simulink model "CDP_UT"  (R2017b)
settings: Solver=FixedStepDiscrete  StartTime=0.0  StopTime=10.0  FixedStep=0.01  RelTol=1e-3  EnableMultiTasking=on
undefined symbols (not defined in the file): ASWTYPE_FALSE, ASWTYPE_TRUE, CaCDP_CellTempNTCVoltTable_mV, CaCDP_CellTempTable_C, CaCDP_CMUPCBTempNTCVoltTable_mV, CaCDP_CMUPCBTempTable_C, CbCDP_DiffBusbarTempStateCheck_flg, CbCDP_DiffCellTempStateCheck_flg, CbCDP_DiffCellVoltStateCheck_flg, CbCDP_IgnorUpdateVld_flg, CbCDP_MaxBusbarTempStateCheck_flg, CbCDP_MaxCellTempStateCheck_flg, CbCDP_MaxCellVoltStateCheck_flg, CbCDP_MinBusbarTempStateCheck_flg, CbCDP_MinCellTempStateCheck_flg, CbCDP_MinCellVoltStateCheck_flg, CcCDP_AFETempConfig_numb, CcCDP_AFETempFltThd_C, CcCDP_AFETempFltThdHys_C, CcCDP_BusbarTempRngFltHiThrd_C, CcCDP_BusbarTempRngFltLowThrd_C, CcCDP_CellDiffFltLevel1_mV, CcCDP_CellDiffFltLevel2_mV, CcCDP_CellDiffFltLevel3_mV, CcCDP_CellTempLowerLimit_C, CcCDP_CellTempRngFltHiThrd_C, CcCDP_CellTempRngFltLowThrd_C, CcCDP_CellTempUpperLimit_C, CcCDP_CellVoltConfig_numb, CcCDP_CellVoltLowerLimit_mV, CcCDP_CellVoltRngHiThrd_mV, CcCDP_CellVoltRngLowThrd_mV, CcCDP_CellVoltUpdateThrd_numb, CcCDP_CellVoltUpperLimit_mV, CcCDP_ChrgMaxCellTempFltLv1Thrd_C, CcCDP_ChrgMaxCellTempFltLv2Thrd_C, CcCDP_ChrgMaxCellTempFltLv3Thrd_C, CcCDP_ChrgMaxCellTempReturnDiff_C, CcCDP_ChrgMinCellTempFltLv1Thrd_C, CcCDP_ChrgMinCellTempFltLv2Thrd_C, CcCDP_ChrgMinCellTempFltLv3Thrd_C, CcCDP_ChrgMinCellTempReturnDiff_C, CcCDP_CMUPCBTempConfig_numb, CcCDP_CMUPCBTempFltThd_C, CcCDP_CMUPCBTempFltThdHys_C, CcCDP_DiffBusbarTempFltLevel1Thrd_C, CcCDP_DiffBusbarTempFltLevel2Thrd_C, CcCDP_DiffBusbarTempReturnDifference_C, CcCDP_DiffCellTempFltLevel1Thrd_C, CcCDP_DiffCellTempFltLevel2Thrd_C, CcCDP_DiffCellTempReturnDifference_C, CcCDP_DiffCellVoltReturnDifference_mV, CcCDP_DiffVoltCheckMaxCellTempCondition_C, CcCDP_DiffVoltCheckMaxCellVoltCondition_mV, CcCDP_DiffVoltCheckMinCellTempCondition_C, CcCDP_DiffVoltCheckMinCellVoltCondition_mV, CcCDP_DiffVoltCheckPackCurrCondition_A, CcCDP_MaxAFETempIniVal_C, CcCDP_MaxBusbarTempFltLevel1Thrd_C, CcCDP_MaxBusbarTempFltLevel2Thrd_C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
libraries: AIWAYS_Powertrain_BMS_lib x148, simulink x8
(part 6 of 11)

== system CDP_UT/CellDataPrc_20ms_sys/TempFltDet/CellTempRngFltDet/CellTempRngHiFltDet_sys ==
  LbCDP_CellTempRngHiChk_flg : Inport
  GcCDP_MaxCellTemp_C : Inport  Port=2
  CDP_GbCDP_ChrgMaxCellVoltFltLv1_flg : AIWAYS_Powertrain_BMS_lib/Signals/OverWrite  OverWrite_Value=CbCDP_CellTempRngHiFltOvr_flg  OverWrite_flag=CbCDP_CellTempRngHiFltOvrSwt_flg
  Constant : Constant  Value=CcCDP_CellTempRngFltHiThrd_C
  Logical Operator1 : Logic  AllPortsSameDT=off  OutDataTypeStr=boolean
  Relational Operator : RelationalOperator  OutDataTypeStr=boolean
  LbCDP_CellTempRngHiFlt_flg : Outport
  GbCDP_CellTempRngHiFlt_flg : Outport  Port=2
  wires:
  GcCDP_MaxCellTemp_C/1 -> Relational Operator/1
  Constant/1 -> Relational Operator/2
  CDP_GbCDP_ChrgMaxCellVoltFltLv1_flg/1 -> GbCDP_CellTempRngHiFlt_flg/1  "GbCDP_CellTempRngHiFlt_flg"
  Logical Operator1/1 -> LbCDP_CellTempRngHiFlt_flg/1, CDP_GbCDP_ChrgMaxCellVoltFltLv1_flg/1  "LbCDP_CellTempRngHiFlt_flg"
  Relational Operator/1 -> Logical Operator1/2
  LbCDP_CellTempRngHiChk_flg/1 -> Logical Operator1/1

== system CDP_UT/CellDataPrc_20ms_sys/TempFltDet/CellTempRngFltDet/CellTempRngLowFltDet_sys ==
  LbCDP_CellTempRngLowChk_flg : Inport
  GcCDP_MinCellTemp_C : Inport  Port=2
  CDP_GbCDP_ChrgMaxCellVoltFltLv1_flg : AIWAYS_Powertrain_BMS_lib/Signals/OverWrite  OverWrite_Value=CbCDP_CellTempRngLowFltOvr_flg  OverWrite_flag=CbCDP_CellTempRngLowFltOvrSwt_flg
  Comparison3 : RelationalOperator  Operator=<=  OutDataTypeStr=boolean
  Constant1 : Constant  Value=CcCDP_CellTempRngFltLowThrd_C
  Logical Operator1 : Logic  AllPortsSameDT=off  OutDataTypeStr=boolean
  LbCDP_CellTempRngLowFlt_flg : Outport
  GbCDP_CellTempRngLowFlt_flg : Outport  Port=2
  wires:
  GcCDP_MinCellTemp_C/1 -> Comparison3/1
  Constant1/1 -> Comparison3/2
  Logical Operator1/1 -> CDP_GbCDP_ChrgMaxCellVoltFltLv1_flg/1, LbCDP_CellTempRngLowFlt_flg/1  "LbCDP_CellTempRngLowFlt_flg"
  CDP_GbCDP_ChrgMaxCellVoltFltLv1_flg/1 -> GbCDP_CellTempRngLowFlt_flg/1  "GbCDP_CellTempRngLowFlt_flg"
  Comparison3/1 -> Logical Operator1/2
  LbCDP_CellTempRngLowChk_flg/1 -> Logical Operator1/1

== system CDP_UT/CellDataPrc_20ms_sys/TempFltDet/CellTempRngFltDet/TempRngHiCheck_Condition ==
  LbCDP_AnyCellTempVld_flg : Inport
  Constant : Constant  Value=ASWTYPE_TRUE
  Constant1 : Constant  Value=CbCDP_MaxCellTempStateCheck_flg
  Constant2 : Constant  Value=ASWTYPE_TRUE
  Logical Operator : Logic  AllPortsSameDT=off  OutDataTypeStr=boolean
  Relational Operator : RelationalOperator  Operator===  OutDataTypeStr=boolean
  Relational Operator1 : RelationalOperator  Operator===  OutDataTypeStr=boolean
  LbCDP_CellTempRngHiChk_flg : Outport
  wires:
  Constant1/1 -> Relational Operator1/1
  Logical Operator/1 -> LbCDP_CellTempRngHiChk_flg/1  "LbCDP_CellTempRngHiChk_flg"
  Relational Operator/1 -> Logical Operator/1
  Constant2/1 -> Relational Operator1/2
  Relational Operator1/1 -> Logical Operator/2
  Constant/1 -> Relational Operator/2
  LbCDP_AnyCellTempVld_flg/1 -> Relational Operator/1

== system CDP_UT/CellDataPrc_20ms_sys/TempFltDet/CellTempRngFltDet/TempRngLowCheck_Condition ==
  LbCDP_AnyCellTempVld_flg : Inport
  Constant : Constant  Value=ASWTYPE_TRUE
  Constant3 : Constant  Value=CbCDP_MinCellTempStateCheck_flg
  Constant4 : Constant  Value=ASWTYPE_TRUE
  Logical Operator : Logic  AllPortsSameDT=off  OutDataTypeStr=boolean
  Relational Operator : RelationalOperator  Operator===  OutDataTypeStr=boolean
  Relational Operator2 : RelationalOperator  Operator===  OutDataTypeStr=boolean
  LbCDP_CellTempRngLowChk_flg : Outport
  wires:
  Relational Operator2/1 -> Logical Operator/2
  Constant3/1 -> Relational Operator2/1
  Constant4/1 -> Relational Operator2/2
  LbCDP_AnyCellTempVld_flg/1 -> Relational Operator/1
  Constant/1 -> Relational Operator/2
  Relational Operator/1 -> Logical Operator/1
  Logical Operator/1 -> LbCDP_CellTempRngLowChk_flg/1  "LbCDP_CellTempRngLowChk_flg"

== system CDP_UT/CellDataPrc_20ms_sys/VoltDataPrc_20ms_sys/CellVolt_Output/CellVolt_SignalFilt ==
  LaCDP_CellVolt_mV : Inport
  LaCDP_CellVoltUpdateVld_flg : Inport  Port=2
  GeUDS_CapSel_enum : Inport  Port=3
  GcUDS_CellVoltNum_numb : Inport  Port=4
  1D_Config_Word : AIWAYS_Powertrain_BMS_lib/Signals/1D_Config_Word  Default_CalPar_Name=CcCDP_CATL203CellVoltFilCfig_numb  CATL153Ah_CalPar_Name=CcCDP_CATL177CellVoltFilCfig_numb  CATL180Ah_CalPar_Name=CcCDP_CATL177CellVoltFilCfig_numb  CATL177Ah_CalPar_Name=CcCDP_CATL177CellVoltFilCfig_numb  CATL203Ah_CalPar_Name=CcCDP_CATL203CellVoltFilCfig_numb  CATL51Ah_CalPar_Name=CcCDP_CATL177CellVoltFilCfig_numb  CATL132Ah_CalPar_Name=CcCDP_CATL177CellVoltFilCfig_numb  XWD75Ah_CalPar_Name=CcCDP_CATL177CellVoltFilCfig_numb  TFE177Ah_CalPar_Name=CcCDP_CATL177CellVoltFilCfig_numb  CATLCTP248Ah_CalPar_Name=CcCDP_CATL177CellVoltFilCfig_numb
  Comparison1 : RelationalOperator  Operator===  OutDataTypeStr=boolean
  Constant2 : Constant  Value=ASWTYPE_FALSE
  InputValueCalc : Stateflow chart  TreatAsAtomicUnit=on
  MaxValue_sort : Stateflow chart  TreatAsAtomicUnit=on
  OverWrite : AIWAYS_Powertrain_BMS_lib/Signals/OverWrite  OverWrite_Value=CaCDP_CellVoltOvr_mV  OverWrite_flag=CbCDP_CellVoltOvrSwt_flg
  SignalDelay1 : Subsystem  Commented=on
  Terminator : Terminator
  Unit Delay21 : UnitDelay  SampleTime=-1  StateName=StateName
  GaCDP_CellVolt_mV : Outport
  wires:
  Unit Delay21/1 -> InputValueCalc/4(Old_Value)
  LaCDP_CellVolt_mV/1 -> InputValueCalc/1(Input_Value)
  MaxValue_sort/2(TargetOutput_Value) -> OverWrite/1
  1D_Config_Word/1 -> MaxValue_sort/2(Input_dim)
  InputValueCalc/1(Output_Value) -> Unit Delay21/1, MaxValue_sort/1(Input_Value)
  GeUDS_CapSel_enum/1 -> 1D_Config_Word/1
  LaCDP_CellVoltUpdateVld_flg/1 -> Comparison1/1
  MaxValue_sort/1(Output_Value) -> Terminator/1
  GcUDS_CellVoltNum_numb/1 -> MaxValue_sort/3(Input_num), InputValueCalc/3(Input_num)
  OverWrite/1 -> GaCDP_CellVolt_mV/1  "GaCDP_CellVolt_mV"
  Constant2/1 -> Comparison1/2
  Comparison1/1 -> InputValueCalc/2(Update)  "LaCDP_CellVoltUpdateVld_flg"

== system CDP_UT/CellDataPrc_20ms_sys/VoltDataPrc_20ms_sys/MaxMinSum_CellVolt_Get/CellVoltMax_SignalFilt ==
  LcCDP_MaxCellVolt_mV : Inport
  LcCDP_MaxCellVoltNumb_numb : Inport  Port=2
  LbCDP_CellVoltUpdateVld_flg : Inport  Port=3
  GeUDS_CapSel_enum : Inport  Port=4
  1D_Config_Word : AIWAYS_Powertrain_BMS_lib/Signals/1D_Config_Word  Default_CalPar_Name=CcCDP_CATL203MaxCellVoltFilCfig_numb  CATL153Ah_CalPar_Name=CcCDP_CATL177MaxCellVoltFilCfig_numb  CATL180Ah_CalPar_Name=CcCDP_CATL177MaxCellVoltFilCfig_numb  CATL177Ah_CalPar_Name=CcCDP_CATL177MaxCellVoltFilCfig_numb  CATL203Ah_CalPar_Name=CcCDP_CATL203MaxCellVoltFilCfig_numb  CATL51Ah_CalPar_Name=CcCDP_CATL177MaxCellVoltFilCfig_numb  CATL132Ah_CalPar_Name=CcCDP_CATL177MaxCellVoltFilCfig_numb  XWD75Ah_CalPar_Name=CcCDP_CATL177MaxCellVoltFilCfig_numb  TFE177Ah_CalPar_Name=CcCDP_CATL177MaxCellVoltFilCfig_numb  CATLCTP248Ah_CalPar_Name=CcCDP_CATL177MaxCellVoltFilCfig_numb
  InputValueCalc : Stateflow chart  TreatAsAtomicUnit=on
  MaxValue_sort : Stateflow chart  TreatAsAtomicUnit=on
  SignalDelay1 : Subsystem  Commented=on
  Unit Delay21 : UnitDelay  SampleTime=-1  StateName=StateName
  ValueCalc : Subsystem
  ValueIndexCalc : Subsystem
  GcCDP_MaxCellVolt_mV : Outport
  GcCDP_MaxCellVoltNumb_numb : Outport  Port=2
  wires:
  ValueCalc/2(Output_index1) -> ValueIndexCalc/1(Output_index1)
  MaxValue_sort/2(Output_index) -> ValueCalc/2(Output_index)
  MaxValue_sort/1(Output_Value) -> ValueCalc/1(Output_Value)
  Unit Delay21/1 -> InputValueCalc/3(Old_Value)
  LcCDP_MaxCellVolt_mV/1 -> InputValueCalc/1(Input_Value)
  LcCDP_MaxCellVoltNumb_numb/1 -> ValueIndexCalc/2(LcCDP_MaxCellVoltNumb_numb)
  ValueIndexCalc/1(GcCDP_MaxCellVoltNumb_numb) -> GcCDP_MaxCellVoltNumb_numb/1
  ValueCalc/1(GcCDP_MaxCellVolt_mV) -> GcCDP_MaxCellVolt_mV/1
  1D_Config_Word/1 -> MaxValue_sort/2(Input_dim), ValueCalc/3(CcCDP_CellVoltFilConfig_numb)
  InputValueCalc/1(Output_Value) -> MaxValue_sort/1(Input_Value), Unit Delay21/1
  GeUDS_CapSel_enum/1 -> 1D_Config_Word/1
  LbCDP_CellVoltUpdateVld_flg/1 -> ValueIndexCalc/3(LbCDP_CellVoltUpdateVld_flg), InputValueCalc/2(Rige)

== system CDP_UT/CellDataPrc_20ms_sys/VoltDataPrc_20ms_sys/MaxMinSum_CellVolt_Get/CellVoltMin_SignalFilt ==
  GeUDS_CapSel_enum : Inport
  LbCDP_CellVoltUpdateVld_flg : Inport  Port=2
  LcCDP_MinCellVolt_mV : Inport  Port=3
  LcCDP_MinCellVoltNumb_numb : Inport  Port=4
  1D_Config_Word : AIWAYS_Powertrain_BMS_lib/Signals/1D_Config_Word  Default_CalPar_Name=CcCDP_CATL203MaxCellVoltFilCfig_numb  CATL153Ah_CalPar_Name=CcCDP_CATL177MaxCellVoltFilCfig_numb  CATL180Ah_CalPar_Name=CcCDP_CATL177MaxCellVoltFilCfig_numb  CATL177Ah_CalPar_Name=CcCDP_CATL177MaxCellVoltFilCfig_numb  CATL203Ah_CalPar_Name=CcCDP_CATL203MaxCellVoltFilCfig_numb  CATL51Ah_CalPar_Name=CcCDP_CATL177MaxCellVoltFilCfig_numb  CATL132Ah_CalPar_Name=CcCDP_CATL177MaxCellVoltFilCfig_numb  XWD75Ah_CalPar_Name=CcCDP_CATL177MaxCellVoltFilCfig_numb  TFE177Ah_CalPar_Name=CcCDP_CATL177MaxCellVoltFilCfig_numb  CATLCTP248Ah_CalPar_Name=CcCDP_CATL177MaxCellVoltFilCfig_numb
  Data Type Conversion : DataTypeConversion
  Data Type Conversion1 : DataTypeConversion
  InputValueCalc : Stateflow chart  TreatAsAtomicUnit=on
  MinValue_sort : Stateflow chart  TreatAsAtomicUnit=on
  SignalDelay1 : Subsystem  Commented=on
  Unit Delay21 : UnitDelay  SampleTime=-1  StateName=StateName
  ValueCalc : Subsystem
  ValueIndexCalc : Subsystem
  GcCDP_MinCellVolt_mV : Outport
  GcCDP_MinCellVoltNumb_numb : Outport  Port=2
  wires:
  1D_Config_Word/1 -> ValueCalc/3(CcCDP_CellVoltFilConfig_numb), Data Type Conversion/1
  GeUDS_CapSel_enum/1 -> 1D_Config_Word/1
  Data Type Conversion1/1 -> MinValue_sort/1(Input_Value)
  Data Type Conversion/1 -> MinValue_sort/2(Input_dim)
  ValueCalc/1(GcCDP_MinCellVolt_mV) -> GcCDP_MinCellVolt_mV/1
  ValueIndexCalc/1(GcCDP_MinCellVoltNumb_numb) -> GcCDP_MinCellVoltNumb_numb/1
  InputValueCalc/1(Output_Value) -> Unit Delay21/1, Data Type Conversion1/1
  LcCDP_MinCellVoltNumb_numb/1 -> ValueIndexCalc/2(LcCDP_MinCellVoltNumb_numb)
  LcCDP_MinCellVolt_mV/1 -> InputValueCalc/1(Input_Value)
  Unit Delay21/1 -> InputValueCalc/3(Old_Value)
  MinValue_sort/1(Output_Value) -> ValueCalc/1(Output_Value)
  MinValue_sort/2(Output_index) -> ValueCalc/2(Output_index)
  ValueCalc/2(Output_index1) -> ValueIndexCalc/1(Output_index1)
  LbCDP_CellVoltUpdateVld_flg/1 -> ValueIndexCalc/3(LbCDP_CellVoltUpdateVld_flg), InputValueCalc/2(Rige)

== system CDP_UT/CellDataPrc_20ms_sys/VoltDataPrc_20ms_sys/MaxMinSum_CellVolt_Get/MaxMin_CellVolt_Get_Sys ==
  LaCDP_CellVoltVld_flg : Inport
  GaISP_CellVoltUpdCnt_numb : Inport  Port=2
  LaCDP_CellVolt_mV : Inport  Port=3
  Enable : EnablePort  StatesWhenEnabling=reset
  Comparison4 : RelationalOperator  Operator===  OutDataTypeStr=boolean
  Constant1 : Constant  Value=CDP_CONST0_NUMB
  Constant2 : Constant  Value=CbCDP_IgnorUpdateVld_flg
  Constant3 : Constant  Value=CcCDP_CellVoltConfig_numb
  Logical : Logic  OutDataTypeStr=boolean
  MaxMin_CellVolt_ForIterator : Subsystem
  Switch : Switch  Criteria=u2 ~= 0  Threshold=1  RndMeth=Zero
  LcCDP_MaxCellVolt_mV : Outport
  LcCDP_MaxCellVoltNumb_numb : Outport  Port=2
  LcCDP_MinCellVolt_mV : Outport  Port=3
  LcCDP_MinCellVoltNumb_numb : Outport  Port=4
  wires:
  LaCDP_CellVolt_mV/1 -> MaxMin_CellVolt_ForIterator/2(LaCDP_CellVolt_mV)
  Constant3/1 -> MaxMin_CellVolt_ForIterator/1(CcCDP_CellVoltConfig_numb)  "CcCDP_CellVoltConfig_numb"
  MaxMin_CellVolt_ForIterator/2(LcCDP_MaxCellVoltNumb_numb) -> LcCDP_MaxCellVoltNumb_numb/1  "LcCDP_MaxCellVoltNumb_numb"
  MaxMin_CellVolt_ForIterator/1(LcCDP_MaxCellVolt_mV) -> LcCDP_MaxCellVolt_mV/1  "LcCDP_MaxCellVolt_mV"
  MaxMin_CellVolt_ForIterator/3(LcCDP_MinCellVolt_mV) -> LcCDP_MinCellVolt_mV/1  "LcCDP_MinCellVolt_mV"
  MaxMin_CellVolt_ForIterator/4(LcCDP_MinCellVoltNumb_numb) -> LcCDP_MinCellVoltNumb_numb/1  "LcCDP_MinCellVoltNumb_numb"
  Comparison4/1 -> Logical/2
  LaCDP_CellVoltVld_flg/1 -> Logical/1, Switch/1
  Logical/1 -> Switch/3
  Constant2/1 -> Switch/2
  Constant1/1 -> Comparison4/2
  GaISP_CellVoltUpdCnt_numb/1 -> Comparison4/1
  Switch/1 -> MaxMin_CellVolt_ForIterator/3(LaCDP_CellVoltVld_flg)

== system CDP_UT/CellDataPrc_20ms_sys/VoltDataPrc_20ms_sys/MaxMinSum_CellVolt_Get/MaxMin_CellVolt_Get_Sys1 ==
  LaCDP_CellVoltVld_flg : Inport
  LaCDP_CellVolt_mV : Inport  Port=2
  Enable : EnablePort  StatesWhenEnabling=reset
  Constant3 : Constant  Value=CcCDP_CellVoltConfig_numb
  MaxMin_CellVolt_ForIterator : Subsystem
  OverWrite : AIWAYS_Powertrain_BMS_lib/Signals/OverWrite  OverWrite_Value=CcCDP_MaxCellVoltOvr_mV  OverWrite_flag=CbCDP_MaxCellVoltOvrSwt_flg
  OverWrite1 : AIWAYS_Powertrain_BMS_lib/Signals/OverWrite  OverWrite_Value=CcCDP_MaxCellVoltNumbOvr_numb  OverWrite_flag=CbCDP_MaxCellVoltNumbOvrSwt_flg
  OverWrite2 : AIWAYS_Powertrain_BMS_lib/Signals/OverWrite  OverWrite_Value=CcCDP_MinCellVoltOvr_mV  OverWrite_flag=CbCDP_MinCellVoltOvrSwt_flg
  OverWrite3 : AIWAYS_Powertrain_BMS_lib/Signals/OverWrite  OverWrite_Value=CcCDP_MinCellVoltNumbOvr_numb  OverWrite_flag=CbCDP_MinCellVoltNumbOvrSwt_flg
  GcCDP_MaxCellVolt_mV : Outport
  GcCDP_MaxCellVoltNumb_numb : Outport  Port=2
  GcCDP_MinCellVolt_mV : Outport  Port=3
  GcCDP_MinCellVoltNumb_numb : Outport  Port=4
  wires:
  LaCDP_CellVoltVld_flg/1 -> MaxMin_CellVolt_ForIterator/3(LaCDP_CellVoltVld_flg)
  MaxMin_CellVolt_ForIterator/4(LcCDP_MinCellVoltNumb_numb) -> OverWrite3/1
  MaxMin_CellVolt_ForIterator/3(LcCDP_MinCellVolt_mV) -> OverWrite2/1
  MaxMin_CellVolt_ForIterator/2(LcCDP_MaxCellVoltNumb_numb) -> OverWrite1/1
  MaxMin_CellVolt_ForIterator/1(LcCDP_MaxCellVolt_mV) -> OverWrite/1
  OverWrite3/1 -> GcCDP_MinCellVoltNumb_numb/1  "GcCDP_MinCellVoltNumb_numb"
  OverWrite2/1 -> GcCDP_MinCellVolt_mV/1  "GcCDP_MinCellVolt_mV"
  OverWrite/1 -> GcCDP_MaxCellVolt_mV/1  "GcCDP_MaxCellVolt_mV"
  OverWrite1/1 -> GcCDP_MaxCellVoltNumb_numb/1  "GcCDP_MaxCellVoltNumb_numb"
  Constant3/1 -> MaxMin_CellVolt_ForIterator/1(CcCDP_CellVoltConfig_numb)  "CcCDP_CellVoltConfig_numb"
  LaCDP_CellVolt_mV/1 -> MaxMin_CellVolt_ForIterator/2(LaCDP_CellVolt_mV)

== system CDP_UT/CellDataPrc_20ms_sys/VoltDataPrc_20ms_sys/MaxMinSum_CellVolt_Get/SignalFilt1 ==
  Input_Value : Inport
  Input_Numb : Inport  Port=2
  GeUDS_CapSel_enum : Inport  Port=3
  1D_Config_Word : AIWAYS_Powertrain_BMS_lib/Signals/1D_Config_Word  Default_CalPar_Name=CcCDP_CATL203CellVoltFilConfig_numb  CATL153Ah_CalPar_Name=CcCDP_CATL177CellVoltFilConfig_numb  CATL180Ah_CalPar_Name=CcCDP_CATL177CellVoltFilConfig_numb  CATL177Ah_CalPar_Name=CcCDP_CATL177CellVoltFilConfig_numb  CATL203Ah_CalPar_Name=CcCDP_CATL203CellVoltFilConfig_numb  CATL51Ah_CalPar_Name=CcCDP_CATL177CellVoltFilConfig_numb  CATL132Ah_CalPar_Name=CcCDP_CATL177CellVoltFilConfig_numb  XWD75Ah_CalPar_Name=CcCDP_CATL177CellVoltFilConfig_numb  TFE177Ah_CalPar_Name=CcCDP_CATL177CellVoltFilConfig_numb  CATLCTP248Ah_CalPar_Name=CcCDP_CATL177CellVoltFilConfig_numb
  Constant2 : Constant  Value=CDP_CONST1_NUMB
  Constant4 : Constant  Value=CDP_CONST2_NUMB
  Constant6 : Constant  Value=CDP_CONST1_NUMB
  Constant7 : Constant  Value=CDP_CONST2_NUMB
  Data Type Conversion : DataTypeConversion
  Data Type Conversion1 : DataTypeConversion
  MaxCellVolt_sort : Stateflow chart  TreatAsAtomicUnit=on
  Product1 : Product  Inputs=*/  OutDataTypeStr=Inherit: Inherit via back propagation
  Product2 : Product  Inputs=*/  OutDataTypeStr=Inherit: Inherit via back propagation
  Selector : Selector  InputPortWidth=5  IndexOptions=Index vector (port)  Indices=[1 3]  OutputSizes=1
  Selector1 : Selector  InputPortWidth=5  IndexOptions=Index vector (port)  Indices=[1 3]  OutputSizes=1
  Selector2 : Selector  IndexMode=Zero-based  InputPortWidth=5  IndexOptions=Index vector (port)  Indices=[1 3]  OutputSizes=1
  SignalDelay1 : Subsystem
  SignalDelay2 : Subsystem
  Sum : Sum  OutDataTypeStr=Inherit: Inherit via back propagation  RndMeth=Zero
  Sum1 : Sum  OutDataTypeStr=Inherit: Inherit via back propagation  RndMeth=Zero
  Output_Value : Outport
  Output_Numb : Outport  Port=2
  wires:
  Input_Value/1 -> SignalDelay1/1(u)
  Input_Numb/1 -> SignalDelay2/1(u)
  SignalDelay1/1(y) -> Data Type Conversion1/1
  MaxCellVolt_sort/1(Output_Value) -> Selector/1
  [CcCDP_CellVoltFilConfig_numb] -> Sum/1
  Constant2/1 -> Sum/2
  Sum/1 -> Product1/1
  Constant4/1 -> Product1/2
  Product1/1 -> Selector/2
  Product2/1 -> Selector1/2
  Constant7/1 -> Product2/2
  Sum1/1 -> Product2/1
  Constant6/1 -> Sum1/2
  [CcCDP_CellVoltFilConfig_numb] -> Sum1/1
  MaxCellVolt_sort/2(Output_index) -> Selector1/1
  SignalDelay2/1(y) -> Selector2/1
  Selector1/1 -> Selector2/2
  Selector2/1 -> Output_Numb/1
  Selector/1 -> Output_Value/1
  Data Type Conversion/1 -> MaxCellVolt_sort/2(Input_dim)
  Data Type Conversion1/1 -> MaxCellVolt_sort/1(Input_Value)
  GeUDS_CapSel_enum/1 -> 1D_Config_Word/1
  1D_Config_Word/1 -> Data Type Conversion/1, [CcCDP_CellVoltFilConfig_numb]

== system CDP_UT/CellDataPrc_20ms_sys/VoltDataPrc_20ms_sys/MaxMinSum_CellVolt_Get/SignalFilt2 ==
  Input_Value : Inport
  Input_Numb : Inport  Port=2
  GeUDS_CapSel_enum : Inport  Port=3
  InputValueVld : Inport  Port=4
  InputValueUpdate : Inport  Port=5
  1D_Config_Word : AIWAYS_Powertrain_BMS_lib/Signals/1D_Config_Word  Default_CalPar_Name=CcCDP_CATL203CellVoltFilConfig_numb  CATL153Ah_CalPar_Name=CcCDP_CATL177CellVoltFilConfig_numb  CATL180Ah_CalPar_Name=CcCDP_CATL177CellVoltFilConfig_numb  CATL177Ah_CalPar_Name=CcCDP_CATL177CellVoltFilConfig_numb  CATL203Ah_CalPar_Name=CcCDP_CATL203CellVoltFilConfig_numb  CATL51Ah_CalPar_Name=CcCDP_CATL177CellVoltFilConfig_numb  CATL132Ah_CalPar_Name=CcCDP_CATL177CellVoltFilConfig_numb  XWD75Ah_CalPar_Name=CcCDP_CATL177CellVoltFilConfig_numb  TFE177Ah_CalPar_Name=CcCDP_CATL177CellVoltFilConfig_numb  CATLCTP248Ah_CalPar_Name=CcCDP_CATL177CellVoltFilConfig_numb
  Bus Creator : BusCreator  Inputs=2
  Bus Selector : BusSelector  OutputSignals=signal1,signal2
  Bus Selector1 : BusSelector  OutputSignals=signal1,signal2
  Comparison4 : RelationalOperator  Operator===  OutDataTypeStr=boolean
  Constant1 : Constant  Value=CDP_CONST0_NUMB
  Data Type Conversion : DataTypeConversion
  Data Type Conversion1 : DataTypeConversion
  EdgeBi : AIWAYS_Powertrain_BMS_lib/Logical Operators/EdgeBi
  InputValueCalc : Stateflow chart  TreatAsAtomicUnit=on
  Logical : Logic  OutDataTypeStr=boolean
  MaxValue_sort : Stateflow chart  TreatAsAtomicUnit=on
  SignalDelay1 : Subsystem  Commented=on
  Unit Delay21 : UnitDelay  SampleTime=-1  StateName=StateName
  ValueCalc : Subsystem
  ValueIndexCalc : Subsystem
  Output_Value : Outport
  Output_Numb : Outport  Port=2
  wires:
  1D_Config_Word/1 -> ValueCalc/3(CcCDP_CellVoltFilConfig_numb), Data Type Conversion/1
  GeUDS_CapSel_enum/1 -> 1D_Config_Word/1
  Data Type Conversion1/1 -> MaxValue_sort/1(Input_Value)
  Data Type Conversion/1 -> MaxValue_sort/2(Input_dim)
  ValueCalc/1(Output_Value1) -> Output_Value/1
  ValueIndexCalc/1(Output_Numb) -> Output_Numb/1
  InputValueCalc/1(Output_Value) -> Unit Delay21/1, Data Type Conversion1/1
  Input_Numb/1 -> ValueIndexCalc/2(Input_Numb)
  Input_Value/1 -> InputValueCalc/1(Input_Value)
  Unit Delay21/1 -> InputValueCalc/3(Old_Value)
  InputValueUpdate/1 -> Bus Creator/2
  Constant1/1 -> Comparison4/2
  InputValueVld/1 -> Bus Creator/1
  Comparison4/1 -> Logical/2
  Logical/1 -> EdgeBi/1
  EdgeBi/1 -> InputValueCalc/2(Rige)
  MaxValue_sort/1(Output_Value) -> ValueCalc/1(Output_Value)
  MaxValue_sort/2(Output_index) -> ValueCalc/2(Output_index)
  ValueCalc/2(Output_index1) -> ValueIndexCalc/1(Output_index1)
  Bus Selector/1 -> Logical/1  "<signal1>"
  Bus Selector/2 -> Comparison4/1  "<signal2>"
  Bus Selector1/1 -> ValueIndexCalc/3(InputValueVld)  "<signal1>"
  Bus Selector1/2 -> ValueIndexCalc/4(InputValueUpdate)  "<signal2>"
  Bus Creator/1 -> Bus Selector1/1, Bus Selector/1

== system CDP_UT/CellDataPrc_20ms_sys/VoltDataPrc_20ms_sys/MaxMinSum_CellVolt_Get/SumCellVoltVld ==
  GaISP_CellVoltUpdCnt_numb : Inport
  LaCDP_CellVoltVld_flg : Inport  Port=2
  CellVoltVld : Subsystem
  Comparison4 : RelationalOperator  Operator===  OutDataTypeStr=boolean
  Constant1 : Constant  Value=CDP_CONST0_NUMB
  Constant2 : Constant  Value=CbCDP_IgnorUpdateVld_flg
  Constant4 : Constant  Value=CcCDP_CellVoltConfig_numb
  Logical : Logic  OutDataTypeStr=boolean
  OverWrite : AIWAYS_Powertrain_BMS_lib/Signals/OverWrite  OverWrite_Value=CbCDP_SumCellVoltVldOvr_flg  OverWrite_flag=CbCDP_SumCellVoltVldOvrSwt_flg
  Switch : Switch  Criteria=u2 ~= 0  Threshold=1  RndMeth=Zero
  GbCDP_SumCellVoltVld_flg : Outport
  LbCDP_SumCellVoltVld_flg : Outport  Port=2
  LbCDP_AnyCellVoltVld_flg : Outport  Port=3
  LbCDP_CellVoltUpdateVld_flg : Outport  Port=4
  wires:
  OverWrite/1 -> GbCDP_SumCellVoltVld_flg/1  "GbCDP_SumCellVoltVld_flg"
  LaCDP_CellVoltVld_flg/1 -> Logical/1, Switch/1
  Constant4/1 -> CellVoltVld/2(CcCDP_CellVoltConfig_numb)
  CellVoltVld/1(LbCDP_AnyCellVoltVld_flg) -> LbCDP_AnyCellVoltVld_flg/1
  CellVoltVld/2(LbCDP_SumCellVoltVld_flg) -> OverWrite/1, LbCDP_SumCellVoltVld_flg/1
  CellVoltVld/3(LbCDP_CellVoltUpdateVld_flg) -> LbCDP_CellVoltUpdateVld_flg/1
  Constant1/1 -> Comparison4/2
  GaISP_CellVoltUpdCnt_numb/1 -> Comparison4/1
  Comparison4/1 -> Logical/2
  Logical/1 -> Switch/3
  Constant2/1 -> Switch/2
  Switch/1 -> CellVoltVld/1(LaCDP_CellVoltVld_flg)

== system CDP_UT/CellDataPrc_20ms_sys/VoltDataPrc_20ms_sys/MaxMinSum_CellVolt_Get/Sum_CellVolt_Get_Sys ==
  LaCDP_CellVolt_mV : Inport
  Enable : EnablePort  StatesWhenEnabling=reset
  Constant3 : Constant  Value=CcCDP_CellVoltConfig_numb
  SumCellVot_Calculation : Subsystem
  Sum_CellVolt_ForIterator : Subsystem
  GcCDP_SumCellVolt_V : Outport
  GcCDP_AvgCellVolt_mV : Outport  Port=2
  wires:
  LaCDP_CellVolt_mV/1 -> Sum_CellVolt_ForIterator/2(LaCDP_CellVolt_mV)
  SumCellVot_Calculation/1(GcCDP_SumCellVolt_V) -> GcCDP_SumCellVolt_V/1
  Sum_CellVolt_ForIterator/1(LcCDP_SumCellVolt_mV) -> SumCellVot_Calculation/1(LcCDP_SumCellVolt_mV)
  Constant3/1 -> Sum_CellVolt_ForIterator/1(CcCDP_CellVoltConfig_numb)  "CcCDP_CellVoltConfig_numb"
  SumCellVot_Calculation/2(GcCDP_AvgCellVolt_mV) -> GcCDP_AvgCellVolt_mV/1

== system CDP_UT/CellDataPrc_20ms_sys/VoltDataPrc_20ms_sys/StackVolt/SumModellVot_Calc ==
  LcCDP_SumModelVolt_mV : Inport
  Constant : Constant  Value=CDP_MV2V_NUMB
  Data Type Conversion : DataTypeConversion
  Divide2 : Product  Inputs=/*  OutDataTypeStr=single
  OverWrite2 : AIWAYS_Powertrain_BMS_lib/Signals/OverWrite  OverWrite_Value=CcCDP_SumModelVoltOvr_V  OverWrite_flag=CbCDP_SumModelVoltOvrSwt_flg
  GcCDP_SumModelVolt_V : Outport
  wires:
  Divide2/1 -> OverWrite2/1
  Constant/1 -> Divide2/1
  OverWrite2/1 -> GcCDP_SumModelVolt_V/1  "GcCDP_SumModelVolt_V"
  LcCDP_SumModelVolt_mV/1 -> Data Type Conversion/1
  Data Type Conversion/1 -> Divide2/2

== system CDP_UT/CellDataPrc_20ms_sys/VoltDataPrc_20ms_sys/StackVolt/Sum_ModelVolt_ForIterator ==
  CcCDP_StackVoltConfig_numb : Inport
  GaISP_StackVolt_mV : Inport  Port=2
  Add : Sum  OutDataTypeStr=Inherit: Inherit via back propagation
  MaxStackVoltNumbIterator : ForIterator  ResetStates=reset  IterationSource=external  IterationVariableDataType=int16
  Selector : Selector  IndexOptions=Index vector (port)  Indices=[1 3]  OutputSizes=1
  Unit Delay : UnitDelay  SampleTime=-1  StateName=StateName
  LcCDP_SumModelVolt_mV : Outport
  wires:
  CcCDP_StackVoltConfig_numb/1 -> MaxStackVoltNumbIterator/1
  MaxStackVoltNumbIterator/1 -> Selector/2
  GaISP_StackVolt_mV/1 -> Selector/1
  Unit Delay/1 -> Add/1
  Add/1 -> LcCDP_SumModelVolt_mV/1, Unit Delay/1  "LcCDP_SumModelVolt_mV"
  Selector/1 -> Add/2

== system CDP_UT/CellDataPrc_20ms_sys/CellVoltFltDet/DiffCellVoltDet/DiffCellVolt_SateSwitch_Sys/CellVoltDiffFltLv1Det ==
  LcCDP_DiffCellVolt_mV : Inport
  LbCDP_DiffvoltCheckCondition_flg : Inport  Port=2
  LbCDP_CellVoltRngLowFlt_flg : Inport  Port=3
  LbCDP_CellVoltRngHiFlt_flg : Inport  Port=4
  Add : Sum  OutDataTypeStr=Inherit: Inherit via back propagation
  Add1 : Sum  OutDataTypeStr=Inherit: Inherit via back propagation
  CDP_GbCDP_ChrgMaxCellVoltFltLv1_flg : AIWAYS_Powertrain_BMS_lib/Signals/OverWrite  OverWrite_Value=CbCDP_CellVoltDiffFltLv1Ovr_flg  OverWrite_flag=CbCDP_CellVoltDiffFltLv1OvrSwt_flg
  Comparison : RelationalOperator  Operator=>  OutDataTypeStr=boolean
  Constant1 : Constant  Value=CcCDP_CellDiffFltLevel1_mV
  Constant2 : Constant  Value=CcCDP_DiffCellVoltReturnDifference_mV
  Constant3 : Constant  Value=CcCDP_CellDiffFltLevel2_mV
  Constant4 : Constant  Value=ASWTYPE_TRUE
  Constant5 : Constant  Value=CcCDP_DiffCellVoltReturnDifference_mV
  Constant6 : Constant  Value=ASWTYPE_FALSE
  Constant7 : Constant  Value=ASWTYPE_FALSE
  Constant8 : Constant  Value=ASWTYPE_TRUE
  Logical Operator : Logic  Inputs=3  AllPortsSameDT=off  OutDataTypeStr=boolean
  Logical Operator1 : Logic  AllPortsSameDT=off  OutDataTypeStr=boolean
  Logical Operator2 : Logic  AllPortsSameDT=off  OutDataTypeStr=boolean
  Relational Operator : RelationalOperator  OutDataTypeStr=boolean
  Relational Operator1 : RelationalOperator  Operator===  OutDataTypeStr=boolean
  Relational Operator2 : RelationalOperator  Operator===  OutDataTypeStr=boolean
  Relational Operator3 : RelationalOperator  Operator===  OutDataTypeStr=boolean
  Terminator : Terminator
  GbCDP_CellVoltDiffFltLv1_flg : Outport
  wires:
  Relational Operator/1 -> Logical Operator1/2
  Constant2/1 -> Add/2
  Constant1/1 -> Add/1
  Add/1 -> Relational Operator/2
  CDP_GbCDP_ChrgMaxCellVoltFltLv1_flg/1 -> GbCDP_CellVoltDiffFltLv1_flg/1  "GbCDP_CellVoltDiffFltLv1_flg"
  Constant4/1 -> Relational Operator1/2
  LbCDP_DiffvoltCheckCondition_flg/1 -> Relational Operator1/1
  Relational Operator1/1 -> Logical Operator/2
  Logical Operator/1 -> CDP_GbCDP_ChrgMaxCellVoltFltLv1_flg/1
  LcCDP_DiffCellVolt_mV/1 -> Relational Operator/1, Comparison/2
  Constant3/1 -> Add1/1
  Constant5/1 -> Add1/2
  Add1/1 -> Comparison/1
  Comparison/1 -> Terminator/1
  Logical Operator1/1 -> Logical Operator/1
  Relational Operator3/1 -> Logical Operator2/2
  LbCDP_CellVoltRngLowFlt_flg/1 -> Relational Operator2/1
  Relational Operator2/1 -> Logical Operator2/1
  LbCDP_CellVoltRngHiFlt_flg/1 -> Relational Operator3/1
  Constant6/1 -> Relational Operator2/2
  Constant7/1 -> Relational Operator3/2
  Logical Operator2/1 -> Logical Operator/3
  Constant8/1 -> Logical Operator1/1

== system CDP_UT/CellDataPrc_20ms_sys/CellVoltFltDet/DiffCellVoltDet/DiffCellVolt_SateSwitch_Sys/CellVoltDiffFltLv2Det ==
  LcCDP_DiffCellVolt_mV : Inport
  LbCDP_DiffvoltCheckCondition_flg : Inport  Port=2
  LbCDP_CellVoltRngLowFlt_flg : Inport  Port=3
  LbCDP_CellVoltRngHiFlt_flg : Inport  Port=4
  Add : Sum  OutDataTypeStr=Inherit: Inherit via back propagation
  Add1 : Sum  OutDataTypeStr=Inherit: Inherit via back propagation
  CDP_GbCDP_ChrgMaxCellVoltFltLv1_flg : AIWAYS_Powertrain_BMS_lib/Signals/OverWrite  OverWrite_Value=CbCDP_CellVoltDiffFltLv2Ovr_flg  OverWrite_flag=CbCDP_CellVoltDiffFltLv2OvrSwt_flg
  Comparison : RelationalOperator  Operator=>  OutDataTypeStr=boolean
  Constant1 : Constant  Value=CcCDP_CellDiffFltLevel2_mV
  Constant2 : Constant  Value=CcCDP_DiffCellVoltReturnDifference_mV
  Constant3 : Constant  Value=CcCDP_CellDiffFltLevel3_mV
  Constant4 : Constant  Value=ASWTYPE_TRUE
  Constant5 : Constant  Value=CcCDP_DiffCellVoltReturnDifference_mV
  Constant6 : Constant  Value=ASWTYPE_FALSE
  Constant7 : Constant  Value=ASWTYPE_FALSE
  Constant8 : Constant  Value=ASWTYPE_TRUE
  Logical Operator : Logic  Inputs=3  AllPortsSameDT=off  OutDataTypeStr=boolean
  Logical Operator1 : Logic  AllPortsSameDT=off  OutDataTypeStr=boolean
  Logical Operator2 : Logic  AllPortsSameDT=off  OutDataTypeStr=boolean
  Relational Operator : RelationalOperator  OutDataTypeStr=boolean
  Relational Operator1 : RelationalOperator  Operator===  OutDataTypeStr=boolean
  Relational Operator2 : RelationalOperator  Operator===  OutDataTypeStr=boolean
  Relational Operator3 : RelationalOperator  Operator===  OutDataTypeStr=boolean
  Terminator : Terminator
  GbCDP_CellVoltDiffFltLv2_flg : Outport
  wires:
  CDP_GbCDP_ChrgMaxCellVoltFltLv1_flg/1 -> GbCDP_CellVoltDiffFltLv2_flg/1  "GbCDP_CellVoltDiffFltLv2_flg"
  Logical Operator/1 -> CDP_GbCDP_ChrgMaxCellVoltFltLv1_flg/1  "LbCDP_CellVoltDiffFltLv2_flg"
  Constant2/1 -> Add/2
  Add/1 -> Relational Operator/2
  LbCDP_DiffvoltCheckCondition_flg/1 -> Relational Operator1/1
  LcCDP_DiffCellVolt_mV/1 -> Relational Operator/1, Comparison/2
  Relational Operator/1 -> Logical Operator1/2
  Logical Operator1/1 -> Logical Operator/1
  Constant4/1 -> Relational Operator1/2
  Add1/1 -> Comparison/1
  Comparison/1 -> Terminator/1
  Constant5/1 -> Add1/2
  Constant1/1 -> Add/1
  Constant3/1 -> Add1/1
  Relational Operator1/1 -> Logical Operator/2
  Relational Operator3/1 -> Logical Operator2/2
  LbCDP_CellVoltRngLowFlt_flg/1 -> Relational Operator2/1
  Relational Operator2/1 -> Logical Operator2/1
  LbCDP_CellVoltRngHiFlt_flg/1 -> Relational Operator3/1
  Constant6/1 -> Relational Operator2/2
  Constant7/1 -> Relational Operator3/2
  Logical Operator2/1 -> Logical Operator/3
  Constant8/1 -> Logical Operator1/1

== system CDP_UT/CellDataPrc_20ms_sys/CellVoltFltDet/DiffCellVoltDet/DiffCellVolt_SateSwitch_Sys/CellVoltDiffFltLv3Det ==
  LcCDP_DiffCellVolt_mV : Inport
  LbCDP_DiffvoltCheckCondition_flg : Inport  Port=2
  LbCDP_CellVoltRngLowFlt_flg : Inport  Port=3
  LbCDP_CellVoltRngHiFlt_flg : Inport  Port=4
  Add : Sum  OutDataTypeStr=Inherit: Inherit via back propagation
  CDP_GbCDP_ChrgMaxCellVoltFltLv1_flg : AIWAYS_Powertrain_BMS_lib/Signals/OverWrite  OverWrite_Value=CbCDP_CellVoltDiffFltLv3Ovr_flg  OverWrite_flag=CbCDP_CellVoltDiffFltLv3OvrSwt_flg
  Constant1 : Constant  Value=CcCDP_CellDiffFltLevel3_mV
  Constant2 : Constant  Value=CcCDP_DiffCellVoltReturnDifference_mV
  Constant3 : Constant  Value=ASWTYPE_TRUE
  Constant4 : Constant  Value=ASWTYPE_FALSE
  Constant5 : Constant  Value=ASWTYPE_FALSE
  Logical Operator : Logic  Inputs=3  AllPortsSameDT=off  OutDataTypeStr=boolean
  Logical Operator1 : Logic  AllPortsSameDT=off  OutDataTypeStr=boolean
  Relational Operator : RelationalOperator  OutDataTypeStr=boolean
  Relational Operator1 : RelationalOperator  Operator===  OutDataTypeStr=boolean
  Relational Operator2 : RelationalOperator  Operator===  OutDataTypeStr=boolean
  Relational Operator3 : RelationalOperator  Operator===  OutDataTypeStr=boolean
  GbCDP_CellVoltDiffFltLv3_flg : Outport
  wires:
  Logical Operator/1 -> CDP_GbCDP_ChrgMaxCellVoltFltLv1_flg/1
  Constant2/1 -> Add/2
  Constant1/1 -> Add/1
  Add/1 -> Relational Operator/2
  LcCDP_DiffCellVolt_mV/1 -> Relational Operator/1
  CDP_GbCDP_ChrgMaxCellVoltFltLv1_flg/1 -> GbCDP_CellVoltDiffFltLv3_flg/1  "GbCDP_CellVoltDiffFltLv3_flg"
  Constant3/1 -> Relational Operator1/2
  LbCDP_DiffvoltCheckCondition_flg/1 -> Relational Operator1/1
  Relational Operator/1 -> Logical Operator/1
  Relational Operator1/1 -> Logical Operator/2
  Constant4/1 -> Relational Operator2/2
  LbCDP_CellVoltRngLowFlt_flg/1 -> Relational Operator2/1
  LbCDP_CellVoltRngHiFlt_flg/1 -> Relational Operator3/1
  Constant5/1 -> Relational Operator3/2
  Relational Operator2/1 -> Logical Operator1/1
  Relational Operator3/1 -> Logical Operator1/2
  Logical Operator1/1 -> Logical Operator/3

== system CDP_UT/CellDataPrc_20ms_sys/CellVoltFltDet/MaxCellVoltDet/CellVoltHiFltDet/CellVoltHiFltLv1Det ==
  LbCDP_MaxVoltCheckCondition_flg : Inport
  GcCDP_MaxCellVolt_mV : Inport  Port=2
  LcCDP_CellHighFltLevel1_mV : Inport  Port=3
  LcCDP_CellHighFltLevel2_mV : Inport  Port=4
  Add1 : Sum  OutDataTypeStr=Inherit: Inherit via back propagation
  Add3 : Sum  OutDataTypeStr=Inherit: Inherit via back propagation
  CDP_GbCDP_ChrgMaxCellVoltFltLv1_flg : AIWAYS_Powertrain_BMS_lib/Signals/OverWrite  OverWrite_Value=CbCDP_CellVoltHiFltLv1Ovr_flg  OverWrite_flag=CbCDP_CellVoltHiFltLv1OvrSwt_flg
  Comparison : RelationalOperator  Operator=>  OutDataTypeStr=boolean
  Constant1 : Constant  Value=CcCDP_MaxCellVoltReturnDifference_mV
  Constant13 : Constant  Value=CcCDP_MaxCellVoltReturnDifference_mV
  Constant2 : Constant  Value=ASWTYPE_TRUE
  Constant3 : Constant  Value=ASWTYPE_TRUE
  Logical Operator : Logic  AllPortsSameDT=off  OutDataTypeStr=boolean
  Logical Operator1 : Logic  AllPortsSameDT=off  OutDataTypeStr=boolean
  Relational Operator1 : RelationalOperator  Operator===  OutDataTypeStr=boolean
  Relational Operator3 : RelationalOperator  OutDataTypeStr=boolean
  Terminator : Terminator
  GbCDP_CellVoltHiFltLv1_flg : Outport
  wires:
  Logical Operator/1 -> CDP_GbCDP_ChrgMaxCellVoltFltLv1_flg/1
  CDP_GbCDP_ChrgMaxCellVoltFltLv1_flg/1 -> GbCDP_CellVoltHiFltLv1_flg/1  "GbCDP_CellVoltHiFltLv1_flg"
  Constant1/1 -> Add1/2
  Comparison/1 -> Terminator/1
  Relational Operator3/1 -> Logical Operator1/2
  LcCDP_CellHighFltLevel1_mV/1 -> Add3/1
  Add3/1 -> Relational Operator3/2
  Constant13/1 -> Add3/2
  Constant2/1 -> Relational Operator1/2
  LbCDP_MaxVoltCheckCondition_flg/1 -> Relational Operator1/1
  LcCDP_CellHighFltLevel2_mV/1 -> Add1/1
  Relational Operator1/1 -> Logical Operator/2
  GcCDP_MaxCellVolt_mV/1 -> Comparison/2, Relational Operator3/1
  Logical Operator1/1 -> Logical Operator/1
  Add1/1 -> Comparison/1
  Constant3/1 -> Logical Operator1/1

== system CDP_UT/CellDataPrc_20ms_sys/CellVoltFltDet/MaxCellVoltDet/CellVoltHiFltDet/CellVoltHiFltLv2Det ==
  LbCDP_MaxVoltCheckCondition_flg : Inport
  GcCDP_MaxCellVolt_mV : Inport  Port=2
  LcCDP_CellHighFltLevel2_mV : Inport  Port=3
  LcCDP_CellHighFltLevel3_mV : Inport  Port=4
  Add1 : Sum  OutDataTypeStr=Inherit: Inherit via back propagation
  Add3 : Sum  OutDataTypeStr=Inherit: Inherit via back propagation
  CDP_GbCDP_ChrgMaxCellVoltFltLv1_flg : AIWAYS_Powertrain_BMS_lib/Signals/OverWrite  OverWrite_Value=CbCDP_CellVoltHiFltLv2Ovr_flg  OverWrite_flag=CbCDP_CellVoltHiFltLv2OvrSwt_flg
  Comparison : RelationalOperator  Operator=>  OutDataTypeStr=boolean
  Constant1 : Constant  Value=CcCDP_MaxCellVoltReturnDifference_mV
  Constant13 : Constant  Value=CcCDP_MaxCellVoltReturnDifference_mV
  Constant2 : Constant  Value=ASWTYPE_TRUE
  Constant3 : Constant  Value=ASWTYPE_TRUE
  Logical Operator : Logic  AllPortsSameDT=off  OutDataTypeStr=boolean
  Logical Operator1 : Logic  AllPortsSameDT=off  OutDataTypeStr=boolean
  Relational Operator1 : RelationalOperator  Operator===  OutDataTypeStr=boolean
  Relational Operator3 : RelationalOperator  OutDataTypeStr=boolean
  Terminator : Terminator
  GbCDP_CellVoltHiFltLv2_flg : Outport
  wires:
  Constant13/1 -> Add3/2
  LcCDP_CellHighFltLevel2_mV/1 -> Add3/1
  Add3/1 -> Relational Operator3/2
  Logical Operator/1 -> CDP_GbCDP_ChrgMaxCellVoltFltLv1_flg/1
  CDP_GbCDP_ChrgMaxCellVoltFltLv1_flg/1 -> GbCDP_CellVoltHiFltLv2_flg/1  "GbCDP_CellVoltHiFltLv2_flg"
  Constant2/1 -> Relational Operator1/2
  LbCDP_MaxVoltCheckCondition_flg/1 -> Relational Operator1/1
  Relational Operator3/1 -> Logical Operator1/2
  Relational Operator1/1 -> Logical Operator/2
  LcCDP_CellHighFltLevel3_mV/1 -> Add1/1
  GcCDP_MaxCellVolt_mV/1 -> Comparison/2, Relational Operator3/1
  Constant1/1 -> Add1/2
  Add1/1 -> Comparison/1
  Comparison/1 -> Terminator/1
  Logical Operator1/1 -> Logical Operator/1
  Constant3/1 -> Logical Operator1/1

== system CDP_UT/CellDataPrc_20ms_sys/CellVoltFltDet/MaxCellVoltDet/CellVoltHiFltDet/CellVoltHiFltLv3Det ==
  LbCDP_MaxVoltCheckCondition_flg : Inport
  GcCDP_MaxCellVolt_mV : Inport  Port=2
  LcCDP_CellHighFltLevel3_mV : Inport  Port=3
  Add3 : Sum  OutDataTypeStr=Inherit: Inherit via back propagation
  CDP_GbCDP_ChrgMaxCellVoltFltLv1_flg : AIWAYS_Powertrain_BMS_lib/Signals/OverWrite  OverWrite_Value=CbCDP_CellVoltHiFltLv3Ovr_flg  OverWrite_flag=CbCDP_CellVoltHiFltLv3OvrSwt_flg
  Comparison : RelationalOperator  Operator=>  OutDataTypeStr=boolean
  Constant1 : Constant  Value=CcCDP_CellVoltRngHiThrd_mV
  Constant13 : Constant  Value=CcCDP_MaxCellVoltReturnDifference_mV
  Constant2 : Constant  Value=ASWTYPE_TRUE
  Constant3 : Constant  Value=ASWTYPE_TRUE
  Logical Operator : Logic  AllPortsSameDT=off  OutDataTypeStr=boolean
  Logical Operator1 : Logic  AllPortsSameDT=off  OutDataTypeStr=boolean
  Relational Operator1 : RelationalOperator  Operator===  OutDataTypeStr=boolean
  Relational Operator3 : RelationalOperator  OutDataTypeStr=boolean
  Terminator : Terminator
  GbCDP_CellVoltHiFltLv3_flg : Outport
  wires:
  Logical Operator/1 -> CDP_GbCDP_ChrgMaxCellVoltFltLv1_flg/1
  CDP_GbCDP_ChrgMaxCellVoltFltLv1_flg/1 -> GbCDP_CellVoltHiFltLv3_flg/1  "GbCDP_CellVoltHiFltLv3_flg"
  Relational Operator3/1 -> Logical Operator1/2
  Constant13/1 -> Add3/2
  GcCDP_MaxCellVolt_mV/1 -> Comparison/2, Relational Operator3/1
  Add3/1 -> Relational Operator3/2
  Logical Operator1/1 -> Logical Operator/1
  Relational Operator1/1 -> Logical Operator/2
  LcCDP_CellHighFltLevel3_mV/1 -> Add3/1
  Comparison/1 -> Terminator/1
  LbCDP_MaxVoltCheckCondition_flg/1 -> Relational Operator1/1
  Constant2/1 -> Relational Operator1/2
  Constant1/1 -> Comparison/1
  Constant3/1 -> Logical Operator1/1

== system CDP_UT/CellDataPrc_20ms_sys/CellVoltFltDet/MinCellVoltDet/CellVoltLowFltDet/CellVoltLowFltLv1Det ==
  LbCDP_MinVoltCheckCondition_flg : Inport
  GcCDP_MinCellVolt_mV : Inport  Port=2
  LcCDP_CellLowFltLevel1_mV : Inport  Port=3
  LcCDP_CellLowFltLevel2_mV : Inport  Port=4
  Add : Sum  Inputs=+-  OutDataTypeStr=Inherit: Inherit via back propagation
  CDP_GbCDP_ChrgMaxCellVoltFltLv1_flg : AIWAYS_Powertrain_BMS_lib/Signals/OverWrite  OverWrite_Value=CbCDP_CellVoltLowFltLv1Ovr_flg  OverWrite_flag=CbCDP_CellVoltLowFltLv1OvrSwt_flg
  Comparison : RelationalOperator  Operator=>  OutDataTypeStr=boolean
  Comparison1 : RelationalOperator  OutDataTypeStr=boolean
  Constant1 : Constant  Value=ASWTYPE_TRUE
  Constant2 : Constant  Value=CcCDP_MinCellVoltReturnDifference_mV
  Constant3 : Constant  Value=ASWTYPE_TRUE
  Logical Operator : Logic  AllPortsSameDT=off  OutDataTypeStr=boolean
  Logical Operator1 : Logic  AllPortsSameDT=off  OutDataTypeStr=boolean
  Relational Operator2 : RelationalOperator  Operator===  OutDataTypeStr=boolean
  Terminator : Terminator
  GbCDP_CellVoltLowFltLv1_flg : Outport
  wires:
  CDP_GbCDP_ChrgMaxCellVoltFltLv1_flg/1 -> GbCDP_CellVoltLowFltLv1_flg/1  "GbCDP_CellVoltLowFltLv1_flg"
  Relational Operator2/1 -> Logical Operator/2
  Constant2/1 -> Add/2
  LbCDP_MinVoltCheckCondition_flg/1 -> Relational Operator2/1
  LcCDP_CellLowFltLevel1_mV/1 -> Add/1
  GcCDP_MinCellVolt_mV/1 -> Comparison1/2, Comparison/1
  LcCDP_CellLowFltLevel2_mV/1 -> Comparison/2
  Comparison1/1 -> Logical Operator1/1
  Add/1 -> Comparison1/1
  Comparison/1 -> Terminator/1
  Logical Operator1/1 -> Logical Operator/1
  Constant1/1 -> Relational Operator2/2
  Logical Operator/1 -> CDP_GbCDP_ChrgMaxCellVoltFltLv1_flg/1
  Constant3/1 -> Logical Operator1/2

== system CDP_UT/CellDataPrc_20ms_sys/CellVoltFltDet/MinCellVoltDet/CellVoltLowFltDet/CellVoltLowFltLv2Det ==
  LbCDP_MinVoltCheckCondition_flg : Inport
  GcCDP_MinCellVolt_mV : Inport  Port=2
  LcCDP_CellLowFltLevel2_mV : Inport  Port=3
  LcCDP_CellLowFltLevel3_mV : Inport  Port=4
  Add : Sum  Inputs=+-  OutDataTypeStr=Inherit: Inherit via back propagation
  CDP_GbCDP_ChrgMaxCellVoltFltLv1_flg : AIWAYS_Powertrain_BMS_lib/Signals/OverWrite  OverWrite_Value=CbCDP_CellVoltLowFltLv2Ovr_flg  OverWrite_flag=CbCDP_CellVoltLowFltLv2OvrSwt_flg
  Comparison : RelationalOperator  Operator=>  OutDataTypeStr=boolean
  Comparison1 : RelationalOperator  OutDataTypeStr=boolean
  Constant1 : Constant  Value=ASWTYPE_TRUE
  Constant2 : Constant  Value=CcCDP_MinCellVoltReturnDifference_mV
  Constant3 : Constant  Value=ASWTYPE_TRUE
  Logical Operator : Logic  AllPortsSameDT=off  OutDataTypeStr=boolean
  Logical Operator1 : Logic  AllPortsSameDT=off  OutDataTypeStr=boolean
  Relational Operator2 : RelationalOperator  Operator===  OutDataTypeStr=boolean
  Terminator : Terminator
  GbCDP_CellVoltLowFltLv2_flg : Outport
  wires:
  Constant2/1 -> Add/2
  Logical Operator/1 -> CDP_GbCDP_ChrgMaxCellVoltFltLv1_flg/1
  LcCDP_CellLowFltLevel2_mV/1 -> Add/1
  Add/1 -> Comparison1/1
  GcCDP_MinCellVolt_mV/1 -> Comparison1/2, Comparison/1
  CDP_GbCDP_ChrgMaxCellVoltFltLv1_flg/1 -> GbCDP_CellVoltLowFltLv2_flg/1  "GbCDP_CellVoltLowFltLv2_flg"
  Constant1/1 -> Relational Operator2/2
  LbCDP_MinVoltCheckCondition_flg/1 -> Relational Operator2/1
  Logical Operator1/1 -> Logical Operator/1
  Relational Operator2/1 -> Logical Operator/2
  LcCDP_CellLowFltLevel3_mV/1 -> Comparison/2
  Comparison1/1 -> Logical Operator1/1
  Comparison/1 -> Terminator/1
  Constant3/1 -> Logical Operator1/2

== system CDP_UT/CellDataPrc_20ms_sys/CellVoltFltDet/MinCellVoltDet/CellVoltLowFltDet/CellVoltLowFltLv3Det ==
  LbCDP_MinVoltCheckCondition_flg : Inport
  GcCDP_MinCellVolt_mV : Inport  Port=2
  LcCDP_CellLowFltLevel3_mV : Inport  Port=3
  Add : Sum  Inputs=+-  OutDataTypeStr=Inherit: Inherit via back propagation
  CDP_GbCDP_ChrgMaxCellVoltFltLv1_flg : AIWAYS_Powertrain_BMS_lib/Signals/OverWrite  OverWrite_Value=CbCDP_CellVoltLowFltLv3Ovr_flg  OverWrite_flag=CbCDP_CellVoltLowFltLv3OvrSwt_flg
  Comparison : RelationalOperator  Operator=>  OutDataTypeStr=boolean
  Comparison1 : RelationalOperator  OutDataTypeStr=boolean
  Constant1 : Constant  Value=ASWTYPE_TRUE
  Constant2 : Constant  Value=CcCDP_MinCellVoltReturnDifference_mV
  Constant3 : Constant  Value=CcCDP_CellVoltRngLowThrd_mV
  Constant4 : Constant  Value=ASWTYPE_TRUE
  Logical Operator : Logic  AllPortsSameDT=off  OutDataTypeStr=boolean
  Logical Operator1 : Logic  AllPortsSameDT=off  OutDataTypeStr=boolean
  Relational Operator2 : RelationalOperator  Operator===  OutDataTypeStr=boolean
  Terminator1 : Terminator
  GbCDP_CellVoltLowFltLv3_flg : Outport
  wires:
  Logical Operator/1 -> CDP_GbCDP_ChrgMaxCellVoltFltLv1_flg/1
  CDP_GbCDP_ChrgMaxCellVoltFltLv1_flg/1 -> GbCDP_CellVoltLowFltLv3_flg/1  "GbCDP_CellVoltLowFltLv3_flg"
  Relational Operator2/1 -> Logical Operator/2
  Constant2/1 -> Add/2
  LbCDP_MinVoltCheckCondition_flg/1 -> Relational Operator2/1
  LcCDP_CellLowFltLevel3_mV/1 -> Add/1
  GcCDP_MinCellVolt_mV/1 -> Comparison1/2, Comparison/1
  Comparison1/1 -> Logical Operator1/1
  Add/1 -> Comparison1/1
  Comparison/1 -> Terminator1/1
  Logical Operator1/1 -> Logical Operator/1
  Constant1/1 -> Relational Operator2/2
  Constant3/1 -> Comparison/2
  Constant4/1 -> Logical Operator1/2

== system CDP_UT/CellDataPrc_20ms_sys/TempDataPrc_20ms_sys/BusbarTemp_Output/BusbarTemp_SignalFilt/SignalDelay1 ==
  u : Inport
  Bus to Vector : BusToVector
  Delay1Cycle : Subsystem
  Delay2Cycle : Subsystem
  Delay3Cycle : Subsystem
  Delay4Cycle : Subsystem
  Mux : Mux  Inputs=5
  y : Outport
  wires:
  u/1 -> Mux/1, Delay4Cycle/1(u), Delay3Cycle/1(u), Delay2Cycle/1(u), Delay1Cycle/1(u)
  Bus to Vector/1 -> y/1
  Delay4Cycle/1(y) -> Mux/5
  Delay2Cycle/1(y) -> Mux/3
  Delay3Cycle/1(y) -> Mux/4
  Delay1Cycle/1(y) -> Mux/2
  Mux/1 -> Bus to Vector/1

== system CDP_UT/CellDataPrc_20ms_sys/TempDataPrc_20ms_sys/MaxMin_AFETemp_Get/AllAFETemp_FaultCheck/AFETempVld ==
  LaCDP_AFETempVld_flg : Inport
  CcCDP_AFETempConfig_numb : Inport  Port=2
  AFETemp : ForIterator  ResetStates=reset  IterationSource=external  IterationVariableDataType=int16
  Logical Operator1 : Logic  Operator=OR  AllPortsSameDT=off  OutDataTypeStr=boolean
  Selector : Selector  IndexOptions=Index vector (port)  Indices=[1 3]  OutputSizes=1
  Unit Delay1 : UnitDelay  SampleTime=-1  StateName=StateName
  LbCDP_AnyAFETempVld_flg : Outport
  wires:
  Unit Delay1/1 -> Logical Operator1/1
  Logical Operator1/1 -> LbCDP_AnyAFETempVld_flg/1, Unit Delay1/1  "LbCDP_AnyAFETempVld_flg"
  LaCDP_AFETempVld_flg/1 -> Selector/1
  CcCDP_AFETempConfig_numb/1 -> AFETemp/1
  AFETemp/1 -> Selector/2
  Selector/1 -> Logical Operator1/2

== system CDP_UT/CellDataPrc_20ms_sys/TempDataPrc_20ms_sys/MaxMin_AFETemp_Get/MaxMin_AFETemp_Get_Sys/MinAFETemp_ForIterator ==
  LaCDP_AFETemp_C : Inport
  LaCDP_AFETempVld_flg : Inport  Port=2
  CcCDP_AFETempConfig_numb : Inport  Port=3
  Bus Creator : BusCreator  Inputs=3
  Bus Selector : BusSelector  OutputSignals=LcCDP_IniOutputAFETemp_C,LcCDP_IniOutputAFETempNumb_numb,LbCDP_IniOutputAFETempVld_flg
  Bus Selector1 : BusSelector  OutputSignals=LcCDP_IniOutputAFETemp_C,LcCDP_IniOutputAFETempNumb_numb,LbCDP_IniOutputAFETempVld_flg
  Data Type Conversion : DataTypeConversion
  MaxAFETemp_ForIterator : Subsystem
  MinAFETempNumbIterator : ForIterator  ResetStates=reset  IterationSource=external  IterationVariableDataType=int8
  MinAFETemp_ForIterator : Subsystem
  Selector1 : Selector  IndexOptions=Index vector (port)  Indices=[1 3]  OutputSizes=1
  Selector2 : Selector  IndexOptions=Index vector (port)  Indices=[1 3]  OutputSizes=1
  LcCDP_MinAFETemp_C : Outport
  LcCDP_MinAFETempNumb_numb : Outport  Port=2
  LcCDP_MaxAFETempNumb_numb : Outport  Port=3
  LcCDP_MaxAFETemp_C : Outport  Port=4
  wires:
  Bus Selector1/3 -> MaxAFETemp_ForIterator/3(LbCDP_IniOutputAFETempVld_flg)  "<LbCDP_IniOutputAFETempVld_flg>"
  Bus Selector/3 -> MinAFETemp_ForIterator/3(LbCDP_IniOutputAFETempVld_flg)  "<LbCDP_IniOutputAFETempVld_flg>"
  Selector2/1 -> Bus Creator/3  "LbCDP_IniOutputAFETempVld_flg"
  LaCDP_AFETempVld_flg/1 -> Selector2/1
  MaxAFETemp_ForIterator/1(LcCDP_MaxAFETempNumb_numb) -> LcCDP_MaxAFETempNumb_numb/1
  MaxAFETemp_ForIterator/2(LcCDP_MaxAFETemp_C) -> LcCDP_MaxAFETemp_C/1
  MinAFETemp_ForIterator/2(LcCDP_MinAFETempNumb_numb) -> LcCDP_MinAFETempNumb_numb/1
  MinAFETemp_ForIterator/1(LcCDP_MinAFETemp_C) -> LcCDP_MinAFETemp_C/1
  Bus Creator/1 -> Bus Selector1/1, Bus Selector/1
  CcCDP_AFETempConfig_numb/1 -> MinAFETempNumbIterator/1
  MinAFETempNumbIterator/1 -> Selector1/2, Data Type Conversion/1, Selector2/2
  LaCDP_AFETemp_C/1 -> Selector1/1
  Selector1/1 -> Bus Creator/1  "LcCDP_IniOutputAFETemp_C"
  Data Type Conversion/1 -> Bus Creator/2  "LcCDP_IniOutputAFETempNumb_numb"
  Bus Selector/1 -> MinAFETemp_ForIterator/1(LcCDP_IniOutputAFETemp_C)  "<LcCDP_IniOutputAFETemp_C>"
  Bus Selector/2 -> MinAFETemp_ForIterator/2(LcCDP_IniOutputAFETempNumb_numb)  "<LcCDP_IniOutputAFETempNumb_numb>"
  Bus Selector1/1 -> MaxAFETemp_ForIterator/1(LcCDP_IniOutputAFETemp_C)  "<LcCDP_IniOutputAFETemp_C>"
  Bus Selector1/2 -> MaxAFETemp_ForIterator/2(LcCDP_IniOutputAFETempNumb_numb)  "<LcCDP_IniOutputAFETempNumb_numb>"

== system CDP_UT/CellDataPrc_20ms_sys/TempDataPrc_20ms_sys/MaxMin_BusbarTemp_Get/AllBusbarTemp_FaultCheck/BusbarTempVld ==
  LaCDP_BusbarTempVld_flg : Inport
  GcUDS_BusbarTempNumb_numb : Inport  Port=2
  BusbarTemp : ForIterator  ResetStates=reset  IterationSource=external  IterationVariableDataType=int16
  Logical Operator : Logic  AllPortsSameDT=off  OutDataTypeStr=boolean
  Logical Operator1 : Logic  Operator=OR  AllPortsSameDT=off  OutDataTypeStr=boolean
  Selector : Selector  IndexOptions=Index vector (port)  Indices=[1 3]  OutputSizes=1
  Unit Delay : UnitDelay  InitialCondition=ASWTYPE_TRUE  SampleTime=-1  StateName=StateName
  Unit Delay1 : UnitDelay  SampleTime=-1  StateName=StateName
  LbCDP_BusbarTempVld_flg : Outport
  LbCDP_AnyBusbarTempVld_flg : Outport  Port=2
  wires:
  Unit Delay1/1 -> Logical Operator1/1
  Logical Operator1/1 -> LbCDP_AnyBusbarTempVld_flg/1, Unit Delay1/1  "LbCDP_AnyBusbarTempVld_flg"
  Unit Delay/1 -> Logical Operator/2
  LaCDP_BusbarTempVld_flg/1 -> Selector/1
  Logical Operator/1 -> LbCDP_BusbarTempVld_flg/1, Unit Delay/1
  GcUDS_BusbarTempNumb_numb/1 -> BusbarTemp/1
  BusbarTemp/1 -> Selector/2
  Selector/1 -> Logical Operator1/2, Logical Operator/1
